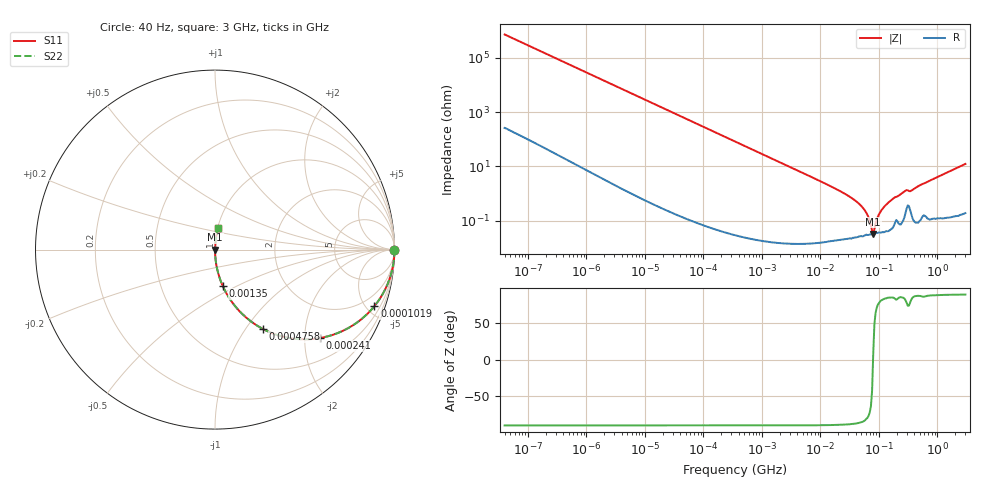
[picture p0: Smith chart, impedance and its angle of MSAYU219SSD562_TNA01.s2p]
! MSAYU219SSD562_TNA01  S-PARAMETER MODEL  ( General Type )
! Model Generated by TAIYO YUDEN Corporation (http://www.ty-top.com)
! Version 2.0
! TAIYO YUDEN Control No. 031016
! Copyright(c) 2003 TAIYO YUDEN CO.,LTD. All Rights Reserved.
! Product Description (link to TY-COMPAS)
! https://ds.yuden.co.jp/TYCOMPAS/or/detail?pn=MSAYU219SSD562KTNA01&u=M
! Products Name : Multilayer Ceramic Capacitors
! Characteristics :
!  Capacitance : 5600 pF , Rated Voltage : 50V
!  Case Size : 2.0 x 1.25 / 0.079 x 0.049 [mm/inch] , Thickness : 0.85 / 0.033 [mm/inch]
!  (Conditions: Temperature = 25 degC , DC Bias Current/Voltage = 0A / 0V)
! External Node Assignments :
!  1  o---| |---o  2
! GND o---------o GND
! Frequency Range : 40Hz  -  3GHz  [ 401 STEP ]
# MHz S RI R 50
! Freq[MHz].  S11 Real  S11 Imag  S21 Real  S21 Imag  S12 Real  S12 Imag  S22 Real  S22 Imag
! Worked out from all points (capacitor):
!   401 points, 40 Hz to 3 GHz, reference 50 ohm
!   read as one part in series: C = 5.55 nF near 44 Hz
!   lowest |Z| = 32.2 mohm at 79.82 MHz (marker M1)
!   series resonance near 79.34 MHz, so ESL is about 720 pH
!   S11 on the Smith chart (normalised r, x): 40 Hz: open; 101.9 kHz: 1.00, -5.63; 241 kHz: 1.00, -2.38; 475.8 kHz: 1.00, -1.20; 1.35 MHz: 1.00, -0.42; 3 GHz: 1.00, +0.25
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4e-05  1 -0.00014  7e-08 0.00014  7e-08 0.00014  1 -0.00014
0.000834  1 -0.00291  9.21e-06 0.00291  9.21e-06 0.00291  1 -0.00291
0.017386  0.9963 -0.0604  0.00368 0.0604  0.00368 0.0604  0.9963 -0.0604
0.045045  0.9759 -0.1533  0.0241 0.1533  0.0241 0.1533  0.9759 -0.1533
0.101865  0.8878 -0.3155  0.1122 0.3155  0.1122 0.3155  0.8878 -0.3155
0.24104  0.5858 -0.4924  0.4142 0.4924  0.4142 0.4924  0.5858 -0.4924
0.362475  0.3848 -0.4864  0.6152 0.4864  0.6152 0.4864  0.3848 -0.4864
0.475778  0.2664 -0.4419  0.7336 0.4419  0.7336 0.4419  0.2664 -0.4419
1.349647  0.0433 -0.2031  0.9567 0.2031  0.9567 0.2031  0.0433 -0.2031
7.222098  0.00169 -0.0393  0.9983 0.0393  0.9983 0.0393  0.00169 -0.0393
23.47158  0.000326 -0.0111  0.9997 0.0111  0.9997 0.0111  0.000326 -0.0111
42.31378  0.000269 -0.00482  0.9997 0.00482  0.9997 0.00482  0.000269 -0.00482
58.11596  0.000294 -0.00226  0.9997 0.00226  0.9997 0.00226  0.000294 -0.00226
66.58224  0.000299 -0.00127  0.9997 0.00127  0.9997 0.00127  0.000299 -0.00127
72.90103  0.000311 -0.000625  0.9997 0.000625  0.9997 0.000625  0.000311 -0.000625
79.8195  0.000319 4.54e-05  0.9997 -4.54e-05  0.9997 -4.54e-05  0.000319 4.54e-05
83.52119  0.000325 0.000364  0.9997 -0.000364  0.9997 -0.000364  0.000325 0.000364
104.7695  0.000365 0.002  0.9996 -0.002  0.9996 -0.002  0.000365 0.002
150.5692  0.000461 0.00495  0.9995 -0.00495  0.9995 -0.00495  0.000461 0.00495
271.4411  0.00143 0.0118  0.9986 -0.0118  0.9986 -0.0118  0.00143 0.0118
356.2883  0.00191 0.0125  0.9981 -0.0125  0.9981 -0.0125  0.00191 0.0125
3000  0.0166 0.1204  0.9834 -0.1204  0.9834 -0.1204  0.0166 0.1204
